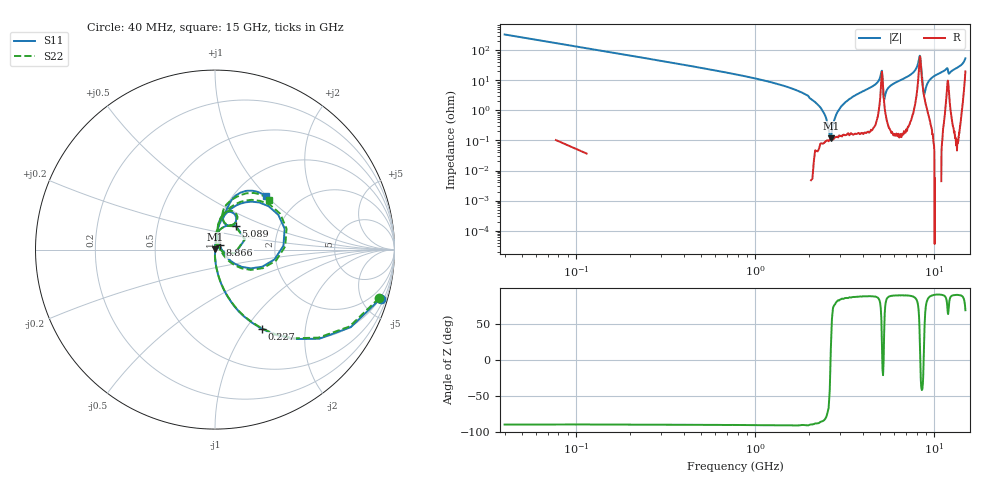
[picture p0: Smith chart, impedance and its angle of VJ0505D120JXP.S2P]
! VJ0505D120JXP
! MLCC placed on 25 mil thick microstrip substrate in series configuraton.
! DATE 06/29/2018  09:01
! CORRECTED  DATA
# GHz  S  MA  R  50.00
!  FREQ  S11M  S11A  S21M  S21A  S12M  S12A  S22M  S22A
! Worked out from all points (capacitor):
!   401 points, 40 MHz to 15 GHz, reference 50 ohm
!   read as one part in series: C = 11.7 pF near 114.8 MHz
!   lowest |Z| = 118 mohm at 2.658 GHz (marker M1)
!   series resonance near 2.649 GHz, so ESL is about 310 pH
!   S11 on the Smith chart (normalised r, x): 40 MHz: 0.93, -6.78; 227 MHz: 0.99, -1.19; 5.089 GHz: 1.21, +0.33; 8.866 GHz: 1.06, +0.05; 15 GHz: 1.38, +0.99
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0.04  0.962 -16.5  0.2831 73.6  0.2834 73.6  0.9536 -16.5
0.227  0.5122 -59.5  0.8606 30.7  0.8609 30.8  0.5078 -59.5
0.601  0.2102 -78.7  0.9787 12.2  0.9791 12.2  0.2085 -78.6
2.0596  0.02249 -91.5  0.9985 1.4  0.9989 1.5  0.02213 -90.9
2.3962  0.007452 -91.0  0.998 0.6  0.9983 0.7  0.007146 -92.5
2.5458  0.001526 -88.0  0.9977 0.3  0.9981 0.4  0.001219 -93.6
2.658  0.00224 81.5  0.9976 0.1  0.9983 0.1  0.002345 86.1
2.7702  0.006352 86.8  0.9975 -0.2  0.998 -0.1  0.006564 90.8
3.1068  0.01743 86.4  0.9971 -0.8  0.9975 -0.7  0.0176 88.3
5.0516  0.1493 64.0  0.9423 -7.8  0.9429 -7.8  0.1465 64.3
5.089  0.1763 48.6  0.8918 -8.1  0.8925 -8.0  0.1733 48.6
5.3134  0.02916 64.7  0.987 -1.2  0.9868 -1.2  0.02794 68.3
5.7622  0.072 84.7  0.9943 -3.7  0.9947 -3.7  0.07104 86.2
7.52  0.163 78.3  0.9795 -9.3  0.9806 -9.2  0.1662 80.0
8.3428  0.4052 16.6  0.617 -10.7  0.6177 -10.7  0.4154 16.3
8.4924  0.226 -27.6  0.8061 7.8  0.8067 7.8  0.2297 -29.5
8.7542  0.04005 -7.1  0.9614 0.3  0.9616 0.4  0.03482 -12.2
8.8664  0.03674 40.7  0.9737 -1.4  0.9745 -1.4  0.03117 47.4
9.2778  0.0842 79.0  0.9875 -4.9  0.9879 -4.9  0.08534 82.0
10.0258  0.135 82.2  0.988 -7.9  0.9894 -7.9  0.1387 82.4
12.5316  0.1888 75.6  0.974 -11.7  0.9749 -11.7  0.195 77.9
15  0.41 46.5  0.77 -23.7  0.7707 -23.7  0.4092 42.5
